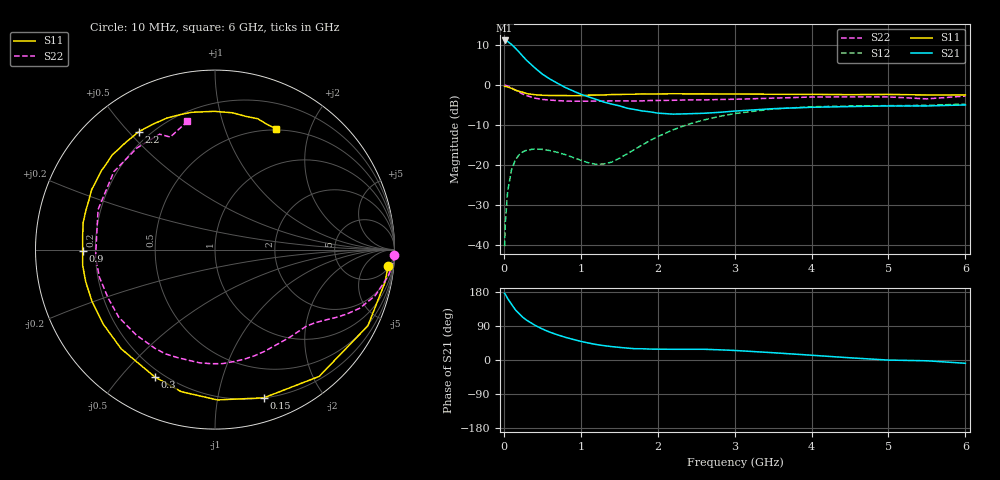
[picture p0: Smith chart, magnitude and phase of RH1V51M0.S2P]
! SIEMENS Small Signal Semiconductors
! BFR106
! Si NPN RF Bipolar Junction Transistor in SOT23
! VCE = 1.5 V  IC = 1 mA
! Common Emitter S-Parameters:  August  1996
# GHz  S  MA  R  50
!  f  S11  S21  S12  S22
! GHz  MAG  ANG  MAG  ANG  MAG  ANG  MAG  ANG
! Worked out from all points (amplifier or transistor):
!   36 points, 10 MHz to 6 GHz, reference 50 ohm
!   highest |S21| = 11.2 dB at 10 MHz (marker M1)
!   |S21| within 3 dB of that: start of sweep to 202.5 MHz
!   unconditionally stable (mu >= 1): 849.4 MHz to end of sweep
!   at 250 MHz: K = 0.28, MSG = 11.9 dB, |S12| = -16.7 dB
!   at 1.4 GHz: K = 1.53, MAG = 3.0 dB, |S12| = -19.3 dB
!   at 6 GHz: K = 1.02, MAG = -1.0 dB, |S12| = -4.7 dB
!   S11 on the Smith chart (normalised r, x): 10 MHz: 6, -19; 150 MHz: 0.20, -1.36; 300 MHz: 0.17, -0.62; 900 MHz: 0.15, -0.00; 2.2 GHz: 0.16, +0.53; 6 GHz: 0.48, +1.51
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0.01  0.9689 -5.4  3.641 175.8  0.0096 88.1  0.9988 -1.8
0.02  0.9646 -10.9  3.641 173.1  0.0193 83.2  0.9977 -3.6
0.05  0.9517 -26.5  3.536 162.0  0.047 74.2  0.9765 -8.7
0.1  0.9143 -50.6  3.248 147.1  0.0874 61.5  0.9281 -16.1
0.15  0.8695 -71.8  2.914 132.5  0.1161 49.6  0.8694 -22.1
0.2  0.8376 -89.1  2.594 122.0  0.1347 41.1  0.8179 -26.0
0.25  0.8136 -103.4  2.287 112.1  0.1469 33.5  0.7712 -29.4
0.3  0.785 -115.2  2.036 104.6  0.1535 28.4  0.7389 -31.8
0.4  0.7608 -133.4  1.662 92.2  0.1588 20.0  0.69 -36.2
0.5  0.7486 -146.4  1.378 81.9  0.157 14.8  0.6635 -40.2
0.7  0.7423 -166.1  1.055 66.3  0.1437 9.4  0.6419 -49.5
0.9  0.7376 -179.5  0.848 54.4  0.1244 10.7  0.63 -59.1
1.1  0.7498 168.4  0.715 44.9  0.1065 19.4  0.6311 -69.8
1.4  0.7639 154.2  0.58 35.4  0.1084 45.5  0.6368 -86.3
1.9  0.7756 133.6  0.464 28.8  0.2026 64.2  0.643 -115.3
2.2  0.7821 123.0  0.434 28.3  0.2762 61.2  0.6472 -132.8
2.8  0.7767 104.8  0.457 26.9  0.4059 47.2  0.6622 -166.7
3.5  0.7704 90.3  0.508 19.2  0.504 29.9  0.6886 161.1
4.5  0.762 76.7  0.54 5.8  0.5489 10.0  0.7141 127.5
5  0.7672 71.9  0.55 -0.2  0.5545 2.9  0.7132 115.6
5.5  0.7545 66.8  0.55 -2.1  0.5594 -0.3  0.6746 111.7
6  0.7552 63.3  0.566 -8.7  0.5798 -7.7  0.731 102.1
